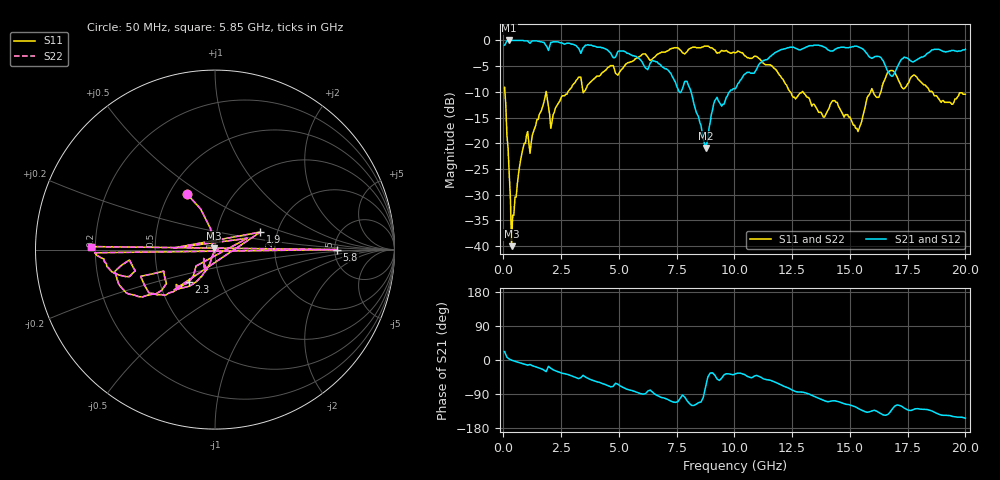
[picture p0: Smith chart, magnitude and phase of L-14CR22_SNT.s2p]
#	mhz	s	ma	r	50
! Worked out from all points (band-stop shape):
!   400 points, 50 MHz to 20 GHz, reference 50 ohm
!   highest |S21| = 0.00 dB at 250 MHz (marker M1); lowest = -20.9 dB at 8.75 GHz (marker M2)
!   |S21| within 3 dB of the highest: start of sweep to 4.703 GHz; 11.59 GHz to 15.81 GHz (4.215 GHz wide, 30.8 % of centre)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
!   lowest |S11| = -40.0 dB at 350 MHz (marker M3), VSWR 1.02, Z = 49.3 + j0.653 ohm
!   |S11| at or under -10 dB: 63.45 MHz to 1.846 GHz (1.782 GHz wide, 187 % of centre); 12.97 GHz to 15.89 GHz (2.922 GHz wide, 20.3 % of centre); 18.57 GHz to end of sweep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
!   |S22| runs from -40.0 to -1.1 dB; largest |S21 - S12| = 0
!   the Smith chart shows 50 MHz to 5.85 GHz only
!   S11 on the Smith chart (normalised r, x): 50 MHz: 0.61, +0.43; 1.9 GHz: 1.63, +0.34; 2.3 GHz: 0.71, -0.27; 5.8 GHz: 5.25, +0.00; 5.85 GHz: 0.18, +0.01
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50  0.35 116.8  0.9 22.2  0.9 22.2  0.35 116.8
250  0.05 103.3  1 2.6  1 2.6  0.05 103.3
350  0.01 138.5  1 -0.4  1 -0.4  0.01 138.5
850  0.09 -110.5  1 -9.8  1 -9.8  0.09 -110.5
1850  0.32 -135.5  0.89 -30.7  0.89 -30.7  0.32 -135.5
1900  0.27 21.1  0.85 -23.6  0.85 -23.6  0.27 21.1
1950  0.23 177.7  0.8 -16.6  0.8 -16.6  0.23 177.7
2000  0.19 19.3  0.88 -19.2  0.88 -19.2  0.19 19.3
2300  0.23 -129.1  0.97 -29.6  0.97 -29.6  0.23 -129.1
3400  0.37 -158.7  0.8 -43.4  0.8 -43.4  0.37 -158.7
5750  0.67 -178.5  0.7 -84.8  0.7 -84.8  0.67 -178.5
5800  0.68 0.0  0.68 -85.8  0.68 -85.8  0.68 0.0
5850  0.69 178.6  0.67 -86.9  0.67 -86.9  0.69 178.6
6700  0.74 167.2  0.6 -94.9  0.6 -94.9  0.74 167.2
7950  0.78 133.7  0.4 -107.5  0.4 -107.5  0.78 133.7
8750  0.88 102.6  0.09 -70.9  0.09 -70.9  0.88 102.6
10050  0.76 85.1  0.34 -36.2  0.34 -36.2  0.76 85.1
11650  0.56 46.6  0.73 -55.6  0.73 -55.6  0.56 46.6
13350  0.23 37.5  0.89 -93.4  0.89 -93.4  0.23 37.5
15350  0.13 34.9  0.87 -127.4  0.87 -127.4  0.13 34.9
16700  0.5 62.4  0.48 -140.0  0.48 -140.0  0.5 62.4
20000  0.3 -53.7  0.82 -153.5  0.82 -153.5  0.3 -53.7
